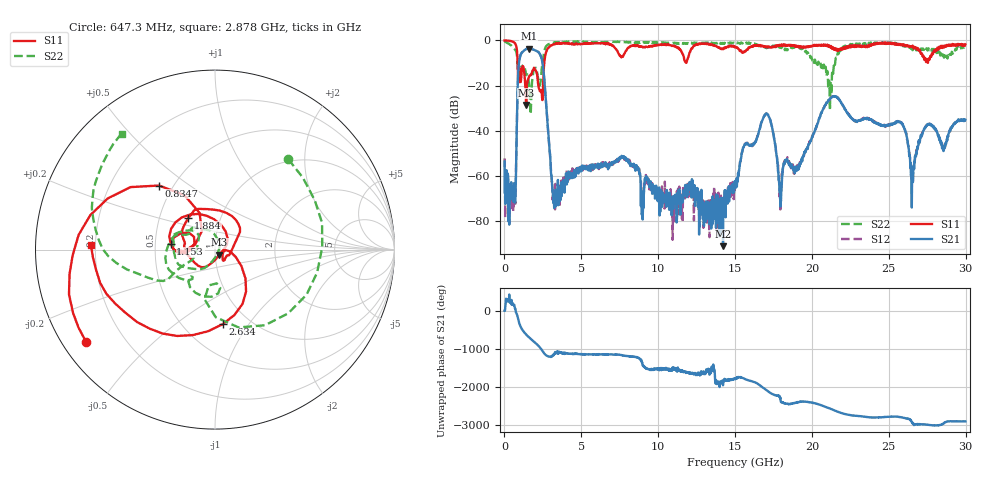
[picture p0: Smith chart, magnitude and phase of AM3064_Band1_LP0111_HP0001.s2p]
# Hz S DB R 50.0
!freq dBS11 angS11 dBS21 angS21 dBS12 angS12 dBS22 angS22
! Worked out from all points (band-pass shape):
!   1600 points, 10 MHz to 29.98 GHz, reference 50 ohm
!   highest |S21| = -3.67 dB at 1.584 GHz (marker M1); lowest = -91.1 dB at 14.22 GHz (marker M2)
!   |S21| within 3 dB of the highest: 1.038 GHz to 2.347 GHz (1.309 GHz wide, 77.3 % of centre)
!   lowest |S11| = -28.6 dB at 1.416 GHz (marker M3), VSWR 1.08, Z = 52.3 - j3.02 ohm
!   |S11| at or under -10 dB: 857.6 MHz to 2.588 GHz (1.73 GHz wide, 100 % of centre)
!   |S22| runs from -32.7 to -0.4 dB; largest |S21 - S12| = 0.011
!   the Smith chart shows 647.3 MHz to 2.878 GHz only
!   S11 on the Smith chart (normalised r, x): 647.3 MHz: 0.07, -0.32; 834.7 MHz: 0.42, +0.39; 1.153 GHz: 0.60, +0.04; 1.884 GHz: 0.70, +0.26; 2.634 GHz: 0.76, -0.76; 2.878 GHz: 0.18, +0.02
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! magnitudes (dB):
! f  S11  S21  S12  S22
! 10 MHz  0.0  -53.7  -52.2  -0.4
! 647.3 MHz  -1.1  -65.0  -66.9  -3.8
! 834.7 MHz  -6.5  -27.3  -27.3  -8.5
! 1.153 GHz  -12.1  -5.3  -5.2  -11.8
! 1.416 GHz  -28.6  -3.8  -3.8  -15.4
! 1.584 GHz  -16.3  -3.7  -3.6  -18.5
! 1.884 GHz  -12.8  -4.1  -4.1  -13.8
! 2.634 GHz  -7.6  -21.1  -21.0  -3.8
! 2.878 GHz  -3.2  -43.6  -43.1  -1.6
! 3.271 GHz  -1.6  -71.2  -68.7  -1.0
! 5.015 GHz  -1.6  -57.0  -55.5  -0.7
! 10 GHz  -2.0  -65.7  -68.4  -0.9
! 14.22 GHz  -3.9  -91.1  -69.8  -1.4
! 15 GHz  -3.0  -65.2  -62.2  -1.4
! 16.99 GHz  -3.0  -32.8  -32.6  -3.1
! 17.93 GHz  -2.0  -67.6  -70.4  -2.6
! 19.99 GHz  -2.7  -43.4  -43.4  -8.1
! 21.42 GHz  -3.8  -24.8  -24.8  -11.1
! 25 GHz  -1.0  -37.3  -37.6  -1.2
! 26.53 GHz  -2.4  -57.8  -59.8  -4.3
! 27.45 GHz  -9.1  -38.0  -37.4  -3.5
! 29.98 GHz  -1.8  -35.1  -35.6  -2.8
